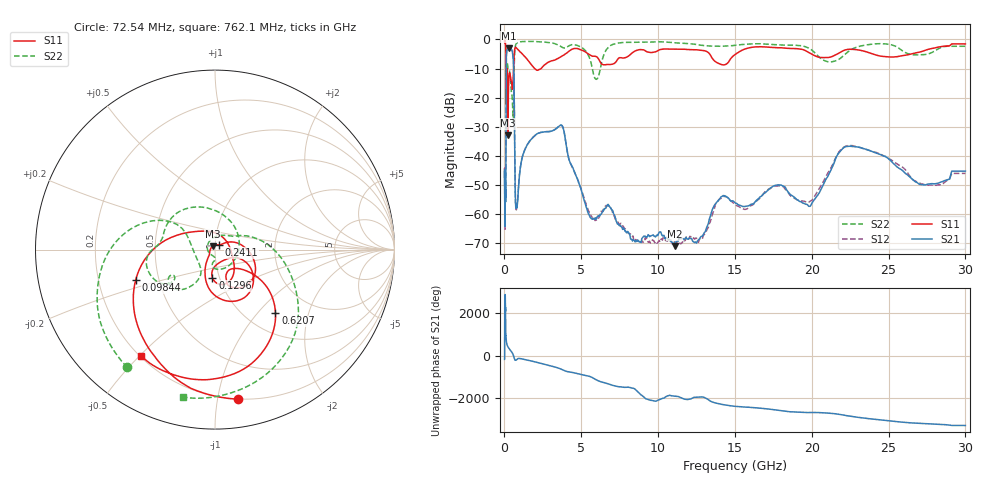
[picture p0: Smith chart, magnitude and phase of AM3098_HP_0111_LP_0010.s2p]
! Date/Time: Thu, Feb 28, 2019 8:38 AM
! Network Analyzer: Agilent Technologies E8364B Rev: A.07.50.67
! Sweep from 0.010 to 30.000 GHz, 1601 Points, Sweep Type: LOG
! Power Supply: 5.022 V, 0.002 A
# Hz S DB R 50
!freq MagS11 AngS11 MagS21 AngS21 MagS12 AngS12 MagS22 AngS22
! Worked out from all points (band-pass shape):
!   1601 points, 10 MHz to 30 GHz, reference 50 ohm
!   highest |S21| = -3.05 dB at 271.8 MHz (marker M1); lowest = -71.1 dB at 11.08 GHz (marker M2)
!   |S21| within 3 dB of the highest: 121 MHz to 563.1 MHz (442.1 MHz wide, 129 % of centre)
!   lowest |S11| = -33.0 dB at 232.8 MHz (marker M3), VSWR 1.05, Z = 48.7 + j1.81 ohm
!   |S11| at or under -10 dB: 102.2 MHz to 588.1 MHz (485.9 MHz wide, 141 % of centre); 1.968 GHz to 2.383 GHz (414.8 MHz wide, 19.1 % of centre)
!   |S22| runs from -28.9 to -0.5 dB; largest |S21 - S12| = 0.011
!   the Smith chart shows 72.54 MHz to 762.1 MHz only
!   S11 on the Smith chart (normalised r, x): 72.54 MHz: 0.20, -1.15; 98.44 MHz: 0.37, -0.16; 129.6 MHz: 0.93, -0.30; 241.1 MHz: 1.05, +0.06; 620.7 MHz: 1.35, -1.25; 762.1 MHz: 0.20, -0.51
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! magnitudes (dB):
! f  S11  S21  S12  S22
! 10 MHz  -0.3  -45.6  -45.5  -0.5
! 38.04 MHz  -0.4  -62.1  -59.5  -0.8
! 72.54 MHz  -1.5  -53.9  -52.8  -1.8
! 86.43 MHz  -2.8  -52.5  -51.9  -2.9
! 98.44 MHz  -6.5  -27.3  -27.3  -7.4
! 129.6 MHz  -16.1  -5.1  -5.1  -10.1
! 144.7 MHz  -20.2  -4.1  -4.1  -11.3
! 186.8 MHz  -11.0  -3.6  -3.6  -8.2
! 232.8 MHz  -33.0  -3.2  -3.2  -9.9
! 241.1 MHz  -29.0  -3.1  -3.1  -10.1
! 271.8 MHz  -15.1  -3.1  -3.0  -10.5
! 550.5 MHz  -15.0  -5.4  -5.4  -25.1
! 620.7 MHz  -6.2  -14.2  -14.2  -12.2
! 762.1 MHz  -2.8  -58.1  -58.2  -1.5
! 2.084 GHz  -10.5  -32.6  -32.5  -0.7
! 3.723 GHz  -5.8  -29.6  -29.5  -2.6
! 5.556 GHz  -5.3  -60.8  -60.3  -6.6
! 7.926 GHz  -6.1  -66.4  -65.7  -1.0
! 11.08 GHz  -3.3  -71.1  -69.9  -1.1
! 19.8 GHz  -4.5  -57.4  -56.0  -3.0
! 22.56 GHz  -3.4  -36.8  -36.5  -3.5
! 30 GHz  -1.5  -45.3  -46.1  -2.3
